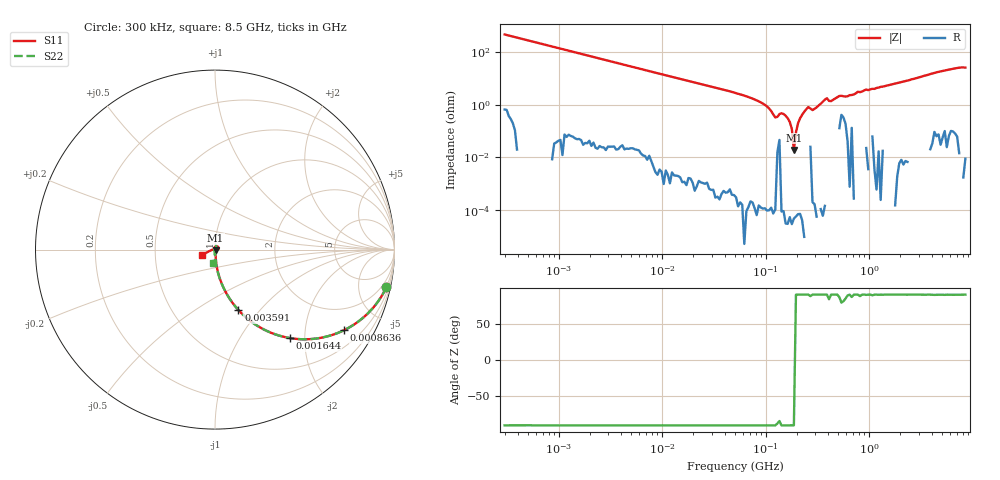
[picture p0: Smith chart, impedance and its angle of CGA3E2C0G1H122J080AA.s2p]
! S-parameter Generated by TDK Corporation
! Copyright(C) 2015 TDK Corporation.
! All Rights Reserved.
! TDK P/N: CGA3E2C0G1H122J080AA (Multilayer Ceramic Chip Capacitors)
! Property: C=1.2nF
! Size(LxWxT): 1.6x0.8x0.8mm, 0.063x0.031x0.031inches
! Model Type: s2p (Touchstone File Format Version 1.0)
! Frequency: DC=Yes Start=0.3MHz Stop=8500MHz 225points Log-sweep
! Note:
! Model Generated on Jun. 23, 2015
! Hash(MD5):
! Port Assignments:
!  1 ---| |--- 2
! Applicable Conditions:
!  Temperature = 25 degC
!  DC Bias Voltage = 0 V
!  Small Signal Operation
! Terms and conditions regarding TDK Simulation Models
! (1)This simulation model is being provided solely for informational purposes. Please refer to the specifications of the products in terms of detailed characteristics of such products.
! (2)In no event shall TDK Corporation of any of its subsidiaries be liable for any loss or damage arising, directly or indirectly,
!  From any information contained in this simulation model, including, but not limited to loss or damages arising from any inaccuracies, omissions or errors in connection with such information.
! (3)Any and all copyrights on this simulation model are owned by TDK Corporation.
!  Duplication or redistribution of this simulation model without prior written permission from TDK Corporation is prohibited.
! (4)This simulation model is subject to any modification or change without any prior notice.
! (5)Neither TDK Corporation nor any of its subsidiaries shall make any warranty, express or implied,
!  Including but not limited to the correctness, implied warranties of merchantability and fitness for a particular purpose with respect to this simulation models.
! (6)The use of this simulation model shall be deemed to have consented to the terms and conditions hereof.
# MHz S MA R 50
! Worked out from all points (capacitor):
!   224 points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, 300 kHz to 8.5 GHz, reference 50 ohm
!   read as one part in series: C = 1.15 nF near 314.1 kHz
!   lowest |Z| = 19 mohm at 187.2 MHz (marker M1)
!   series resonance near 188.7 MHz, so ESL is about 620 pH
!   S11 on the Smith chart (normalised r, x): 300 kHz: 0.99, -9.13; 863.6 kHz: 1.00, -3.21; 1.644 MHz: 1.00, -1.69; 3.591 MHz: 1.00, -0.77; 8.5 GHz: 0.87, -0.05
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0.3  0.9771 -12.4  0.2126 77.5  0.2126 77.7  0.9771 -12.4
0.8636283  0.8485 -31.9  0.528 58.1  0.5282 58.1  0.8482 -31.9
1.643778  0.6454 -49.8  0.7637 40.2  0.7637 40.2  0.6453 -49.8
1.72111  0.628 -51.1  0.7781 38.9  0.7781 38.9  0.628 -51.1
3.591337  0.3613 -68.8  0.9323 21.1  0.9324 21.2  0.3613 -68.8
9.430415  0.1476 -81.4  0.989 8.4  0.989 8.5  0.1476 -81.7
51.67171  0.02846 -82.5  0.9996 1.5  0.9996 1.5  0.02846 -94.4
187.1913  0.004942 -52.5  1 -0.2  1 -0.2  0.004942 -127.9
283.1228  0.001538 -136.1  1 -0.8  1 -0.8  0.001538 -45.5
324.9909  0.0005689 -13.4  1 -1.1  1 -1.1  0.0005689 -168.7
390.6008  0.006363 96.6  1 -1.7  1 -1.6  0.006363 80.1
408.9767  0.003219 48.7  0.9985 -1.5  0.9983 -1.5  0.001294 48.8
538.8791  0.008158 62.6  0.9957 -2.1  0.9956 -2.1  0.005548 37.3
710.042  0.001642 105.2  1 -2.7  1 -2.7  0.001642 69.4
778.4218  0.00496 106.6  1 -3.3  1 -3.3  0.00496 66.8
815.0429  0.003864 74.4  0.9986 -3.3  0.9985 -3.3  0.001222 66.1
935.5712  0.006457 125.9  0.9996 -4.1  0.9996 -3.9  0.006325 39.6
1551.304  0.004284 120.7  1 -6.2  1 -6.1  0.004284 47.1
2819.992  0.003381 165.8  1 -11.6  1 -11.4  0.003381 -8.9
4895.91  0.02275 53.1  0.9993 -20.2  0.9992 -20.1  0.02277 84.3
7072.242  0.0068 33.5  0.9986 -29.2  0.9983 -29.1  0.00384 93.6
8500  0.07554 -157.4  0.9941 -35.1  0.9937 -35.1  0.07615 -97.6
